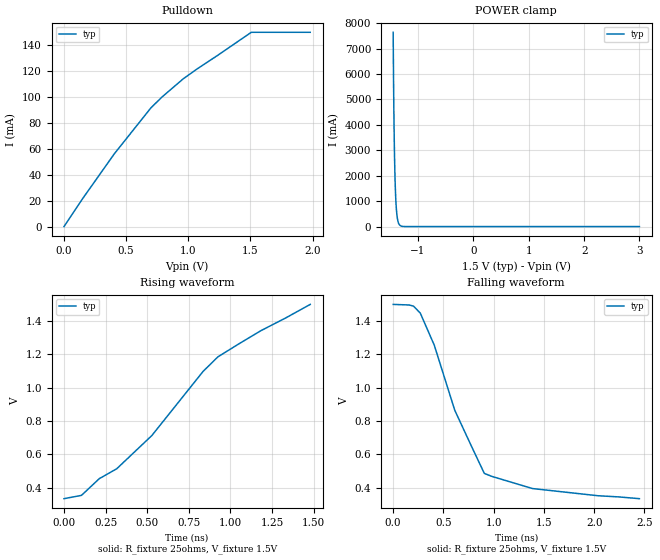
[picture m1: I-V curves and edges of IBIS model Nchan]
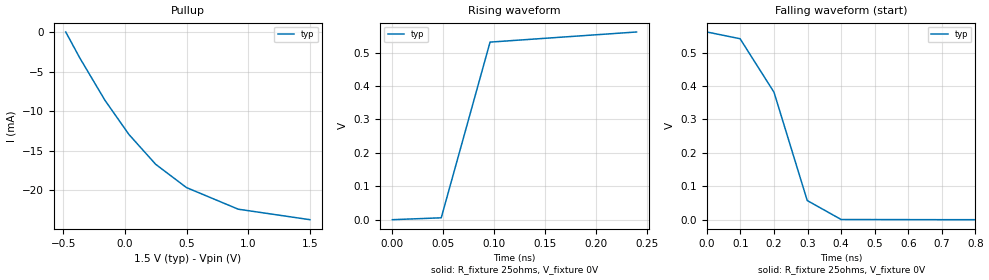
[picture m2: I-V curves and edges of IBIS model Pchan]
[IBIS Ver]	2.1
[File Name]	aardvark.ibs
[File Rev]	0.1
[Source]
[Date]		4/7/97
[Comment char]	|_char
|  The following model demonstrates the use of IBIS multistage driver
|  schedules to describe an inverting and non-inverting model
|  with pulsed turn-off of the pullup transistor in an output
|  stage.  In this example, during pullup cycles the pullup driver
|  is turned on at time=0 and then turned off at time=10ns.  The pulldown
|  driver is always on during the pulldown part of the cycle.
[Component]	aardvark
[Manufacturer]	Manufacturer Name
[Package]
| variable 	typ	min	max
R_pkg		0ohms	NA	NA
L_pkg		0H	NA	NA
C_pkg		0F	NA	NA
[Pin]   signal_name   model_name   R_pin   L_pin   C_pin
1	1		10ns_Non-Inverting
2	2		10ns_Inverting
[Package Model] aardvarkPackage_long
[Define Package Model]  aardvarkPackage_long
[Manufacturer]
[Number of Sections]   4
[Number of Pins]   2
[Pin Numbers]
1   Len=0 L=4n  / Len=0.52 L=11.46n c=2.95p R=0.26 / Len=0.33 L=10.36n C=3.25p R=0.26 / Len=0 L=0.34n /
2   Len=0 L=4n  / Len=0.52 L=11.46n c=2.95p R=0.26 / Len=0.33 L=10.36n C=3.25p R=0.26 / Len=0 L=0.34n /
[End Package Model]
[Model]	10ns_Non-Inverting
Model_type  I/O
Polarity   Non-Inverting
Enable   Active-Low
Vinl = 0.9
Vinh = 1.1
Vmeas = 1.00
Cref  = 0.00p
Rref  = 25.00
Vref  = 1.50
| variable	typ	min	max
C_comp		3.28pF	NA	NA
[Voltage Range]	1.5V	NA	NA
[Driver Schedule]
|	Model_name	Rise_on_dly	Rise_off_dly	Fall_on_dly	Fall_off_dly
	Nchan 		0		NA		0		NA
	Pchan 		0		10n		NA		NA
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[Ramp]
| variable	typ	min	max
dV/dt_r	631.08mV/1.86ns	NA	NA
dV/dt_f	631.08mV/1.86ns	NA	NA
R_load = 25ohms
[Model]	10ns_Inverting
Model_type  I/O
Polarity   Inverting
Enable   Active-Low
Vinl = 0.9
Vinh = 1.1
Vmeas = 1.00
Cref  = 0.00p
Rref  = 25.00
Vref  = 1.50
| variable	typ	min	max
C_comp		3.28pF	NA	NA
[Voltage Range]	1.5V	NA	NA
[Driver Schedule]
|	Model_name	Rise_on_dly	Rise_off_dly	Fall_on_dly	Fall_off_dly
	Nchan 		0		NA		0		NA
	Pchan 		0		10n		NA		NA
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[Ramp]
| variable	typ	min	max
dV/dt_r	631.08mV/1.86ns	NA	NA
dV/dt_f	631.08mV/1.86ns	NA	NA
R_load = 25ohms
| Models and submodels in the file (4): 10ns_Non-Inverting (I/O), 10ns_Inverting (I/O), Nchan (I/O_open_drain), Pchan (I/O)
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[Model]	Nchan
Model_type  I/O_open_drain
Polarity   Non-Inverting
Enable   Active-Low
Vinl = 0.9
Vinh = 1.1
Vmeas = 1.00
Cref  = 0.00p
Rref  = 25.00
Vref  = 1.50
| variable	typ	min	max
C_comp		3.28pF	NA	NA
[Voltage Range]	1.5V	NA	NA
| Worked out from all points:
|   slope of the pulldown table from 0 to 0.225 V, typ, clamps not added: 7.08 ohm
|   POWER clamp passes 1 mA (typ) near -1.23 V on its own axis
|   rising waveform, R_fixture 25ohms, V_fixture 1.5V: 20-80 % time 683ps typ, NA min, NA max; typ from 0.334 V to 1.5 V
|   falling waveform, R_fixture 25ohms, V_fixture 1.5V: 20-80 % time 442ps typ, NA min, NA max; typ from 1.5 V to 0.334 V
[POWER Clamp]
|Voltage	I(typ)	I(min)	I(max)   Table is VCC relative
-1.45V    7.64A      NA         NA
-1.443V   5.72A      NA         NA
-1.437V   4.46A      NA         NA
-1.431V   3.48A      NA         NA
-1.425V   2.71A      NA         NA
-1.418V   2.03A      NA         NA
-1.412V   1.58A      NA         NA
-1.397V   850mA      NA         NA
-1.379V   400mA      NA         NA
-1.354V   140mA      NA         NA
-1.321V   36.66mA    NA         NA
2.998V    0A         NA         NA
[Pullup]
|Voltage	I(typ)	I(min)	I(max)   Table is VCC relative
-481mV    0A         NA         NA
-480mV    0A         NA         NA
1.499V    0A         NA         NA
[Pulldown]
|Voltage	I(typ)	I(min)	I(max)
0V        0A         NA         NA
150mV     21.59mA    NA         NA
406mV     56.34mA    NA         NA
699mV     91.6mA     NA         NA
788mV     100mA      NA         NA
962mV     114.3mA    NA         NA
1.07V     121.6mA    NA         NA
1.237V    132.3mA    NA         NA
1.507V    150mA      NA         NA
1.981V    150mA      NA         NA
[Ramp]
| variable	typ	min	max
dV/dt_r	698.4mV/888ps	NA	NA
dV/dt_f	698.4mV/1.47ns	NA	NA
R_load = 25ohms
[Rising Waveform]
R_fixture = 25ohms
V_fixture = 1.5V
|Time	V(typ)	V(min)	V(max)
0s        334.2mV    NA         NA
105ps     354mV      NA         NA
212ps     454.1mV    NA         NA
317ps     513.4mV    NA         NA
528ps     712.5mV    NA         NA
836ps     1.097V     NA         NA
925ps     1.184V     NA         NA
1.184ns   1.341V     NA         NA
1.48ns    1.498V     NA         NA
[Falling Waveform]
R_fixture = 25ohms
V_fixture = 1.5V
|Time	V(typ)	V(min)	V(max)
0s        1.498V     NA         NA
159ps     1.495V     NA         NA
203ps     1.488V     NA         NA
270ps     1.446V     NA         NA
409ps     1.254V     NA         NA
613ps     863.8mV    NA         NA
907ps     485.5mV    NA         NA
1.387ns   394.7mV    NA         NA
2.041ns   351.6mV    NA         NA
2.45ns    334.2mV    NA         NA
[Model] Pchan
Model_type  I/O
Polarity   Non-Inverting
Enable   Active-Low
Vinl = 0.9
Vinh = 1.1
Vmeas = 1.00
Cref  = 0.00p
Rref  = 25.00
Vref  = 1.50
| variable	typ	min	max
C_comp		3.28pF	NA	NA
[Voltage Range]	1.5V	NA	NA
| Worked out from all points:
|   slope of the pullup table from 0 to 0.225 V, typ, clamps not added: 55.2 ohm
|   rising waveform, R_fixture 25ohms, V_fixture 0V: 20-80 % time 30.8ps typ, NA min, NA max; typ from 0 V to 0.562 V
|   falling waveform, R_fixture 25ohms, V_fixture 0V: 20-80 % time 125ps typ, NA min, NA max; typ from 0.562 V to 0 V
[Pullup]
|Voltage	I(typ)	I(min)	I(max)   Table is VCC relative
-481mV    32uA       NA         NA
-479mV    -28uA      NA         NA
-368mV    -3.23mA    NA         NA
-163mV    -8.62mA    NA         NA
32mV      -12.96mA   NA         NA
249mV     -16.74mA   NA         NA
499mV     -19.69mA   NA         NA
919mV     -22.43mA   NA         NA
1.501V    -23.76mA   NA         NA
[Pulldown]
|Voltage	I(typ)	I(min)	I(max)
0V        0A         NA         NA
2V        0A         NA         NA
[Ramp]
| variable	typ	min	max
dV/dt_r	337.09mV/144ps	NA	NA
dV/dt_f	337.09mV/1.32ns	NA	NA
R_load = 25ohms
[Rising Waveform]
R_fixture = 25ohms
V_fixture = 0V
|Time	V(typ)	V(min)	V(max)
0s        -22.89uV   NA         NA
48ps      5.6mV      NA         NA
96ps      531.5mV    NA         NA
240ps     561.8mV    NA         NA
[Falling Waveform]
R_fixture = 25ohms
V_fixture = 0V
|Time	V(typ)	V(min)	V(max)
0s        561.8mV    NA         NA
99ps      541.6mV    NA         NA
200ps     381.5mV    NA         NA
299ps     57.28mV    NA         NA
400ps     538.9uV    NA         NA
700ps     -22.89uV   NA         NA
2.101ns   -22.89uV   NA         NA
2.2ns     -22.89uV   NA         NA
